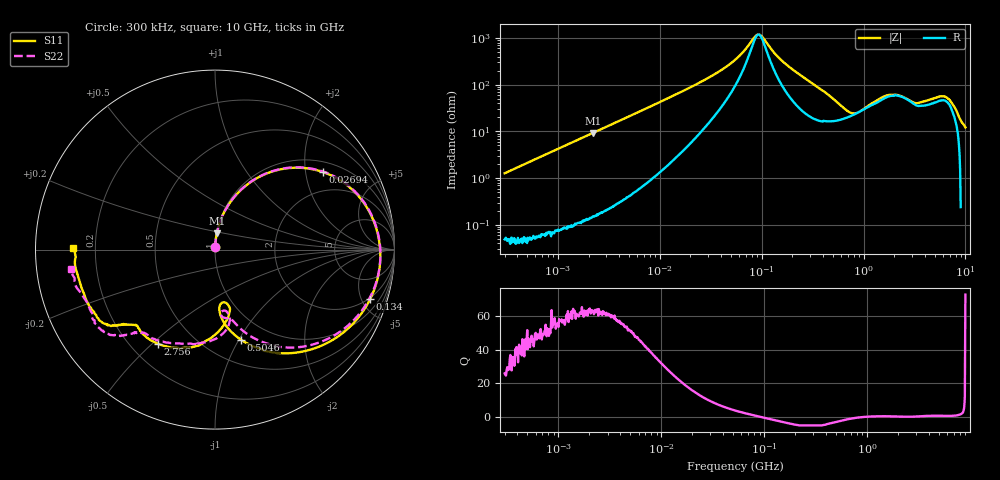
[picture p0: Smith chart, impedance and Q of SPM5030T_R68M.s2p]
! S-Parameter Data Generated by TDK Corporation
! Copyright(C) 2024 TDK Corporation.
! All Rights Reserved.
! TDK P/N: SPM5030T-R68M (SMD / SMT Inductor (Coil))
! Property: L=680nH at 100kHz
! Size(LxWxT): 5.2x5x3mm
! Model Type: s2p (Touchstone File Format Version 1.0)
! Frequency: DC=Yes Start=0.3MHz Stop=10000MHz 802points Log-sweep
! Model Generated on May 28, 2024
! Terms and conditions regarding TDK Simulation Models:
! 1)This simulation model is being provided solely for informational
!  purposes. Please refer to the specifications of the products in
!  terms of detailed characteristics of such products.
! 2)In no event shall TDK Corporation of any of its subsidiaries be
!  liable for any loss or damage arising, directly or indirectly,
!  from any information contained in this simulation model, including,
!  but not limited to loss or damages arising from any inaccuracies,
!  omissions or errors in connection with such information.
! 3)Any and all copyrights on this simulation model are owned by
!  TDK Corporation.  Duplication or redistribution of this simulation
!  model without prior written permission from TDK Corporation
!  is prohibited.
! 4)This simulation model is subject to any modification or change
!  without any prior notice.
! 5)Neither TDK Corporation nor any of its subsidiaries shall make any
!  warranty, express or implied, including but not limited to the
!  correctness, implied warranties of merchantability and fitness for
!  a particular purpose with respect to this simulation models.
! 6)The use of this simulation model shall be deemed to have consented
!  to the terms and conditions hereof.
! Port Assignments:
!  1 ---@@@--- 2
! Applicable Conditions:
!  Temperature = 25 degC
!  DC Bias Current = 0 A
!  Small Signal Operation
# Hz S MA R 50
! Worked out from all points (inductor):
!   801 points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, 300 kHz to 10 GHz, reference 50 ohm
!   read as one part in series: L = 673 nH near 318.3 kHz
!   highest Q = 63.4 at 2.211 MHz (marker M1), where L = 670 nH
!   self-resonance near 93.37 MHz
!   S11 on the Smith chart (normalised r, x): 300 kHz: 1.00, +0.03; 26.94 MHz: 1.31, +2.51; 134 MHz: 1.88, -5.85; 504.6 MHz: 0.74, -1.02; 2.756 GHz: 0.31, -0.52; 10 GHz: 0.12, +0.00
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300000  0.01253 86.4  0.9995 -0.8  0.9993 -0.7  0.01242 87.7
1713600  0.07112 84.9  0.9962 -4.2  0.9964 -4.2  0.07108 84.9
2211197  0.0916 83.6  0.9942 -5.4  0.9943 -5.4  0.0916 83.7
9671944  0.3719 65.9  0.9168 -22.3  0.917 -22.3  0.3719 66.0
1.740512e7  0.5845 50.2  0.7801 -36.6  0.7803 -36.6  0.5845 50.4
2.693747e7  0.7411 35.6  0.6064 -48.9  0.6066 -48.9  0.7412 36.0
5.477226e7  0.8936 11.6  0.2649 -61.9  0.265 -61.9  0.8936 12.4
9.209736e7  0.9226 -4.9  0.07761 -8.8  0.07764 -8.8  0.9226 -3.6
1.014901e8  0.9217 -8.1  0.08702 19.8  0.08706 19.8  0.9218 -6.6
1.340254e8  0.9074 -17.7  0.1896 49.3  0.1897 49.3  0.9078 -15.7
2.013356e8  0.8478 -33.6  0.382 46.1  0.3821 46.1  0.8491 -30.5
3.126428e8  0.7189 -53.3  0.5842 29.9  0.5843 29.9  0.7236 -48.5
5.046115e8  0.5227 -73.9  0.7245 6.6  0.7246 6.6  0.5403 -66.1
7.235338e8  0.3826 -84.5  0.7491 -13.2  0.7492 -13.2  0.4266 -74.6
1.069912e9  0.2978 -81.9  0.6672 -35.9  0.6673 -35.9  0.3843 -81.9
1.323741e9  0.3496 -76.3  0.6096 -45.0  0.6097 -45.0  0.345 -80.4
1.767019e9  0.4704 -89.4  0.4913 -62.1  0.4913 -62.1  0.5015 -90.8
2.756092e9  0.6139 -121.4  0.3885 -74.1  0.3887 -74.2  0.5844 -117.6
3.429941e9  0.6063 -135.1  0.3751 -91.0  0.3748 -91.0  0.6067 -129.5
4.22443e9  0.6475 -139.7  0.2927 -111.7  0.2925 -111.8  0.6558 -134.5
6.333834e9  0.7532 -148.1  0.155 -131.7  0.1549 -131.9  0.7714 -143.6
1e10  0.7886 179.5  0.09518 -154.2  0.09545 -154.0  0.8123 -172.3
